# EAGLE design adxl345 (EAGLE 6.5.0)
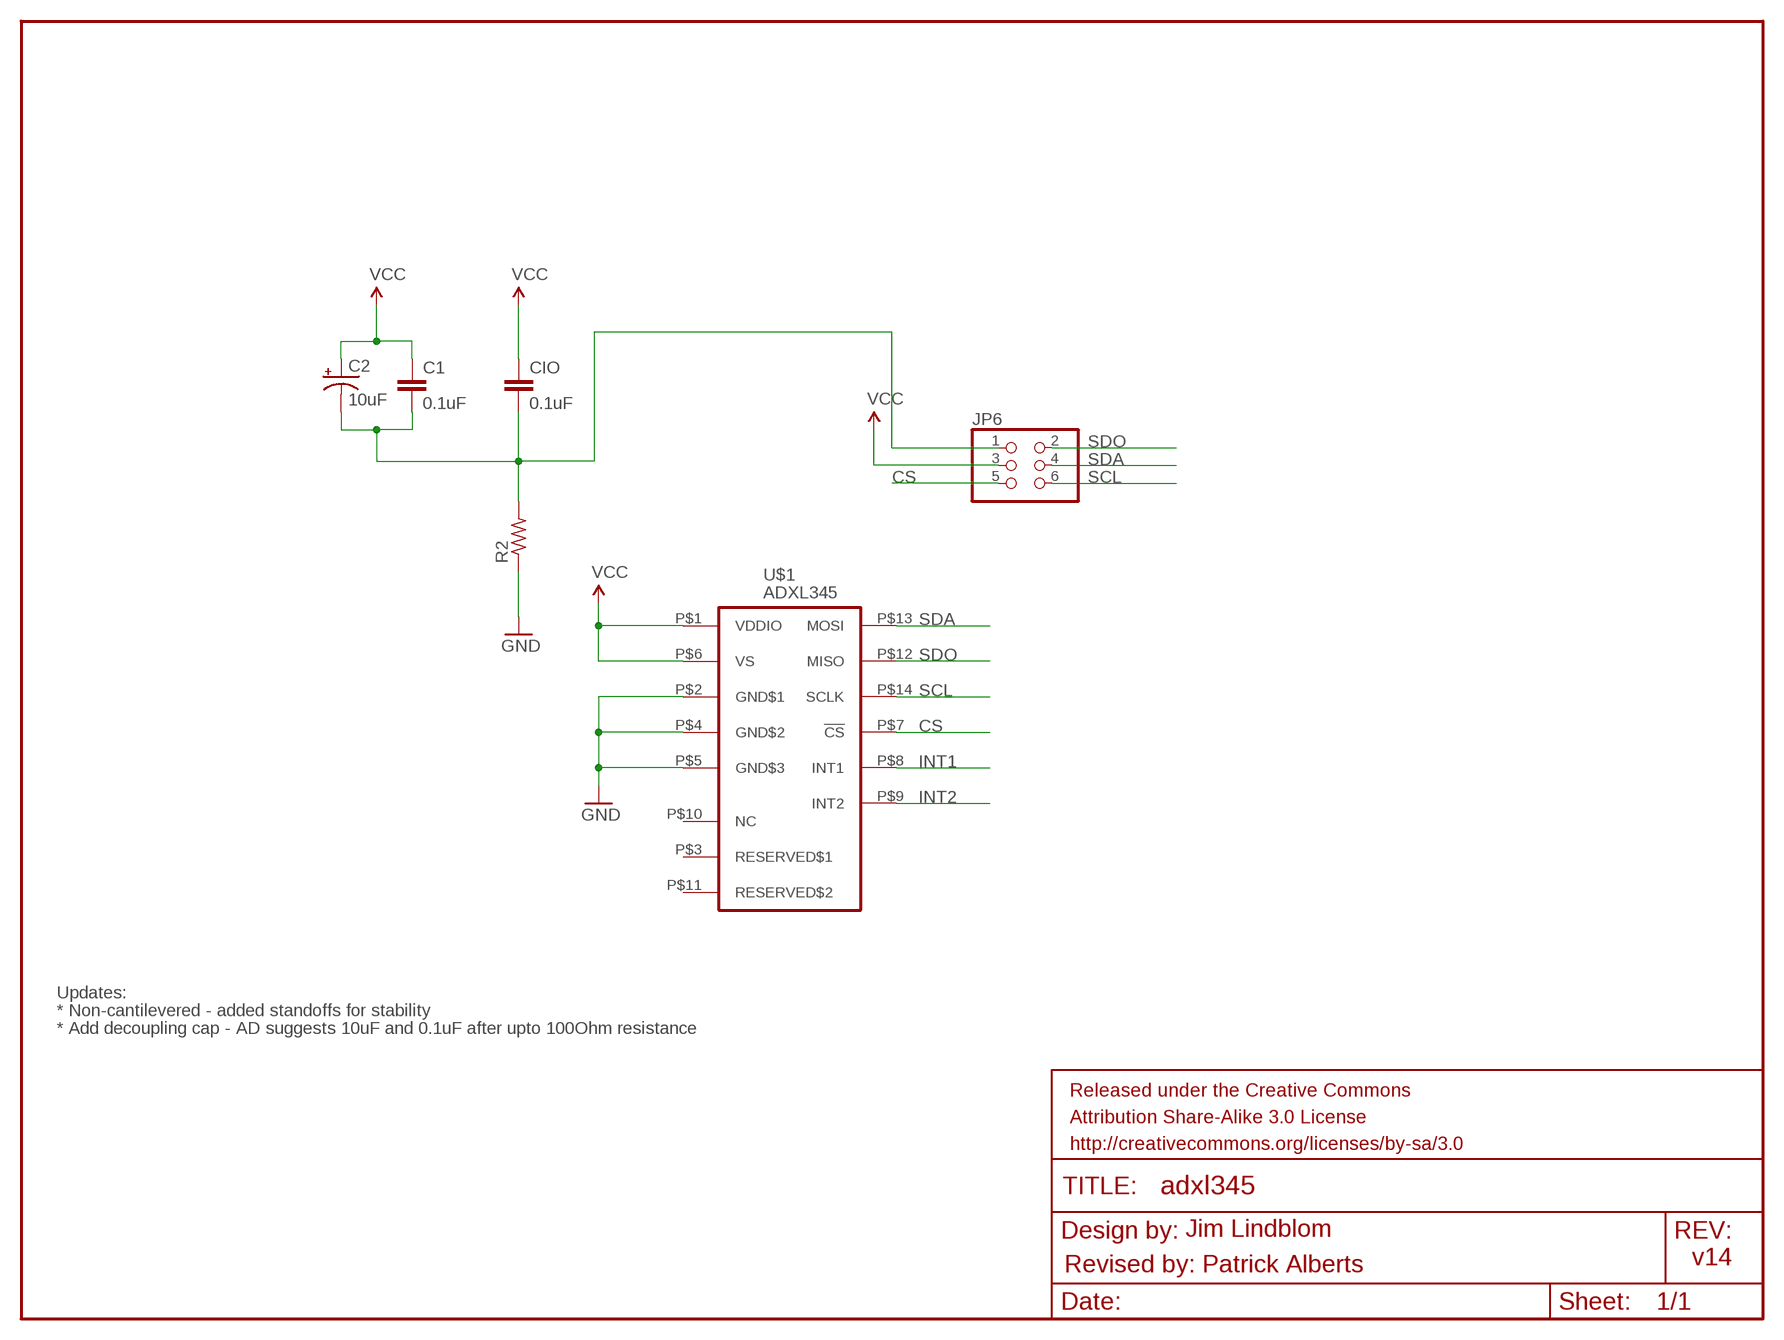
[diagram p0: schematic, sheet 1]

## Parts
C1  0.1uF  CAP0603-CAP  [0603-CAP]
C2  10uF  CAP_POL1206  [EIA3216]
CIO  0.1uF  CAP0603-CAP  [0603-CAP]
JP6  PINHD-2X3-SMD  [2X03SMD]
R2  RESISTOR1206  [1206]
U$1  ADXL345  [LGA14]

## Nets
CS: JP6.5 U$1.P$7(!CS)
GND: R2.1 U$1.P$2(GND$1) U$1.P$4(GND$2) U$1.P$5(GND$3)
INT1: U$1.P$8(INT1)
INT2: U$1.P$9(INT2)
N$1: C1.2 C2.C(-) CIO.2 JP6.1 R2.2
SCL: JP6.6 U$1.P$14(SCLK)
SDA: JP6.4 U$1.P$13(MOSI)
SDO: JP6.2 U$1.P$12(MISO)
VCC: C1.1 C2.A(+) CIO.1 JP6.3 U$1.P$1(VDDIO) U$1.P$6(VS)
Unconnected: U$1.P$3(RESERVED$1) U$1.P$10(NC) U$1.P$11(RESERVED$2)

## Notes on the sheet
- Updates:
- * Non-cantilevered - added standoffs for stability
- * Add decoupling cap - AD suggests 10uF and 0.1uF after upto 100Ohm resistance
- Jim Lindblom
- v14
- Revised by: Patrick Alberts

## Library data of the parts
C1 CIO = SparkFun:CAP: Capacitor
C2 = SparkFun:CAP_POL: Capacitor Polarized
JP6 = fab:PINHD-2X3-SMD: PIN HEADER
R2 = ng:RESISTOR
U$1 = leek:ADXL345: 3-Axis, ±2 g/±4 g/±8 g/±16 g Digital Accelerometer

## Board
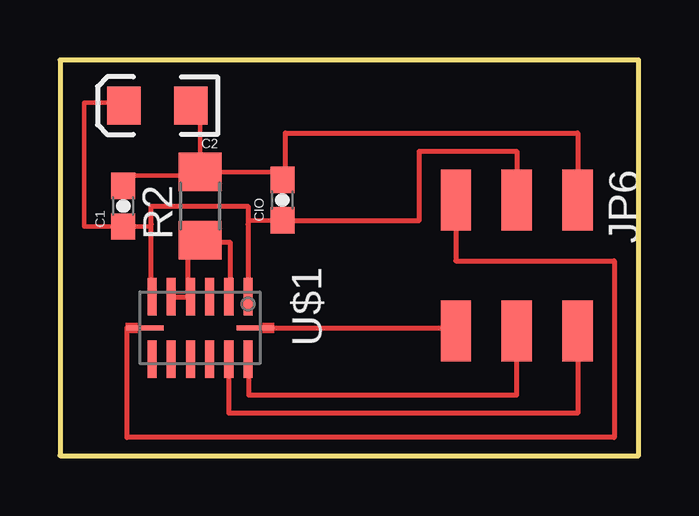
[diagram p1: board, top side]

Size 24.13 x 16.51 mm. Coordinates in mm from the lower left corner, seen from the top.
Outline: 0,0 24.13,0 24.13,16.51 0,16.51 0,0
Copper layers (1*16): Top 0.035mm / dielectric 1.5mm / Bottom 0.035mm
Design rules "SparkFun *": minimum track width 8mil, minimum drill 20mil, track to track 16mil, track to pad 16mil, pad to pad 16mil, via to via 16mil, smd to smd 16mil, copper to edge 16mil, drill to drill 16mil, minimum pad ring 12mil, minimum via ring 10mil, stop-mask expansion 4mil, vias tented up to drill 20mil, thermal gap 10mil

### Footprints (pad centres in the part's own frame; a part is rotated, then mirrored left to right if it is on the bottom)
0603-CAP = smd 1.1 x 1: 1 -0.85,0; 2 0.85,0
EIA3216 = smd 1.4 x 1.6: A 1.4,0; C -1.4,0
2X03SMD = smd 2.54 x 1.27: 1 -2.54,2.54; 2 2.92,2.54; 3 -2.54,0; 4 2.92,0; 5 -2.54,-2.54; 6 2.92,-2.54
1206 = smd 1.6 x 1.803: 1 -1.422,0; 2 1.422,0
LGA14 = smd 1.55 x 0.38: P$1 -1.3,2; P$2 -1.3,1.2; P$3 -1.3,0.4; P$4 -1.3,-0.4; P$5 -1.3,-1.2; P$6 -1.3,-2; P$8 1.3,-2; P$9 1.3,-1.2; P$10 1.3,-0.4; P$11 1.3,0.4; P$12 1.3,1.2; P$13 1.3,2 | smd 0.2 x 1.55: P$7 0,-2.3; P$14 0,2.3

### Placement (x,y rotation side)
C1  2.64,10.41 90 top
C2  4.06,14.61 180 top
CIO  9.27,10.67 90 top
JP6  19.05,8.13 270 top
R2  5.84,10.41 90 top
U$1  5.84,5.33 270 top

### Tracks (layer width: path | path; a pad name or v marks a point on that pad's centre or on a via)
CS
  Top 0.203: JP6.5 16.51,8.13 23.11,8.13 23.11,0.76 2.79,0.76 2.79,5.33 U$1.P$7
GND
  Top 0.203: U$1.P$5 U$1.P$4 5.33,6.63 5.33,8.89 5.84,8.89 | U$1.P$2 7.11,6.63 7.11,8.89 5.84,8.89 | 5.84,8.89 R2.1
N$1
  Top 0.178: 5.84,11.68 2.64,11.68 C1.2 | C2.C 5.84,14.61 R2.2 9.27,11.84 CIO.2
  Top 0.203: 5.84,11.68 R2.2 | CIO.2 9.4,11.52 9.4,13.46 21.59,13.46 JP6.1
SCL
  Top 0.178: U$1.P$14 8.64,5.33
  Top 0.203: 8.64,5.33 16.51,5.33 JP6.6
SDA
  Top 0.203: U$1.P$13 7.87,4.03 7.87,2.54 19.05,2.54 JP6.4
SDO
  Top 0.203: JP6.2 21.59,1.78 7.04,1.78 U$1.P$12
VCC
  Top 0.178: 3.81,9.65 3.81,9.56 C1.1 1.02,9.56 1.02,14.73 2.66,14.73 C2.A | CIO.1 7.84,9.82 7.84,9.65
  Top 0.203: U$1.P$1 7.84,9.65 7.84,10.41 3.81,10.41 3.81,9.65 3.81,6.63 U$1.P$6 3.84,6.6 | CIO.1 14.99,9.82 14.99,12.7 19.05,12.7 JP6.3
